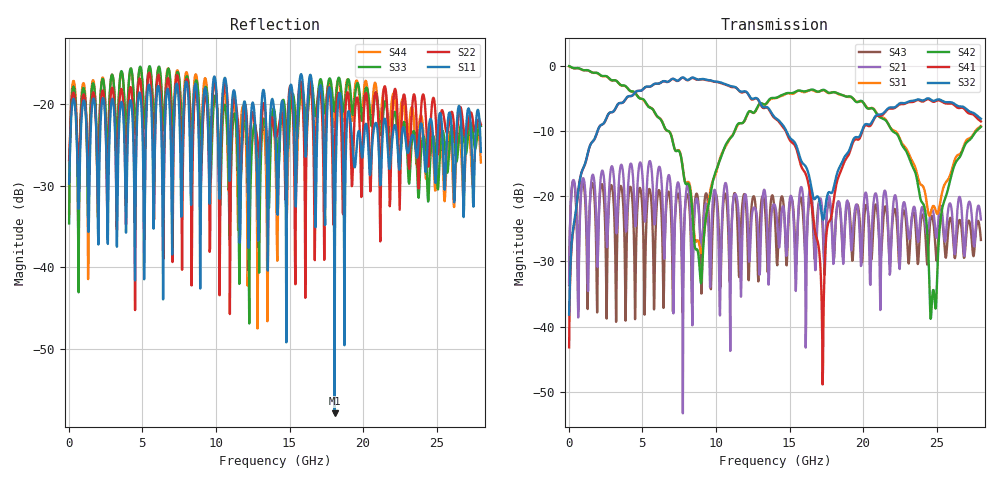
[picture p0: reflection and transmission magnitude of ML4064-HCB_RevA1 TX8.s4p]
! TOUCHSTONE file generated by CST DESIGN STUDIO
! Date and time: Wed Aug 26 10:56:07 2020
! Project name:  Project name: C:\Users\Simulation2\Temp\DE66\Untitled_0.cst
! Tree item: Tasks\SPara1\S-Parameters
# GHz S MA R 50
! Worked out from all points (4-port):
!   1000 points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, 28 MHz to 28 GHz, reference 50 ohm
!   strongest paths, dB at 28 MHz, 7.028 GHz, 14.03 GHz, 21.03 GHz, 28 GHz:
!     S32: -38.2, -2.0, -8.0, -7.5, -8.1
!     S41: -43.2, -2.0, -8.1, -7.7, -8.5
!     S42: -0.1, -11.3, -4.9, -7.7, -9.4
!     S31: -0.1, -11.2, -5.0, -7.7, -9.2
!     S21: -33.6, -24.1, -21.5, -23.0, -23.6
!     S43: -33.1, -29.2, -24.0, -24.1, -26.7
!   lowest |S11| = -57.9 dB at 18.06 GHz (marker M1), VSWR 1.00, Z = 49.9 + j0.0837 ohm
!   |S11| at or under -10 dB: start of sweep to end of sweep
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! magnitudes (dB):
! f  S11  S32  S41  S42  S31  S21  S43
! 28 MHz  -29.7  -38.2  -43.2  -0.1  -0.1  -33.6  -33.1
! 2.072 GHz  -28.6  -9.4  -9.4  -1.3  -1.3  -21.2  -21.5
! 8.96 GHz  -35.8  -2.1  -2.1  -33.1  -28.4  -26.8  -29.1
! 17.22 GHz  -19.2  -23.2  -41.5  -3.7  -3.8  -22.1  -23.4
! 18.06 GHz  -57.9  -18.1  -19.8  -4.1  -4.1  -27.2  -28.1
! 24.72 GHz  -23.3  -5.4  -5.5  -34.7  -21.6  -22.1  -23.4
! 28 GHz  -25.8  -8.1  -8.5  -9.4  -9.2  -23.6  -26.7
